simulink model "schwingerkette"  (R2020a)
settings: Solver=ode45  StartTime=0.0  StopTime=10.0  RelTol=1e-3  EnableMultiTasking=on

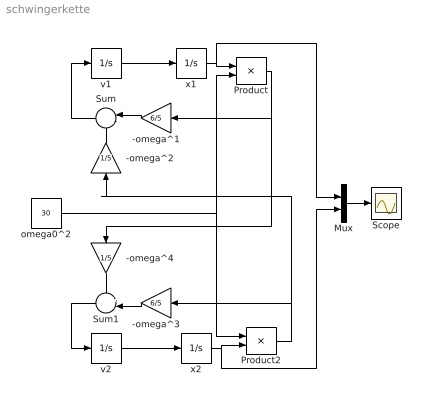
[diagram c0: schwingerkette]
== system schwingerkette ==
  -omega^1 : Gain  Gain=6/5  SaturateOnIntegerOverflow=on
  -omega^2 : Gain  Gain=1/5  SaturateOnIntegerOverflow=on
  -omega^3 : Gain  Gain=6/5  SaturateOnIntegerOverflow=on
  -omega^4 : Gain  Gain=1/5  SaturateOnIntegerOverflow=on
  Mux : Mux  Inputs=2
  Product : Product  InputSameDT=on  RndMeth=Zero  SaturateOnIntegerOverflow=on
  Product2 : Product  InputSameDT=on  RndMeth=Zero  SaturateOnIntegerOverflow=on
  Scope : Scope
  Sum : Sum  Inputs=|-+  InputSameDT=on  SaturateOnIntegerOverflow=on
  Sum1 : Sum  Inputs=+-|  InputSameDT=on  SaturateOnIntegerOverflow=on
  omega0^2 : Constant  Value=30
  v1 : Integrator
  v2 : Integrator
  x1 : Integrator  InitialCondition=1
  x2 : Integrator
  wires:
  v1/1 -> x1/1
  Mux/1 -> Scope/1
  v2/1 -> x2/1
  x1/1 -> Product/1, Mux/1
  x2/1 -> Product2/2, Mux/2
  omega0^2/1 -> Product/2, Product2/1
  -omega^2/1 -> Sum/2
  -omega^1/1 -> Sum/1
  Product/1 -> -omega^1/1, -omega^4/1
  Sum/1 -> v1/1
  Product2/1 -> -omega^2/1, -omega^3/1
  -omega^3/1 -> Sum1/2
  -omega^4/1 -> Sum1/1
  Sum1/1 -> v2/1
